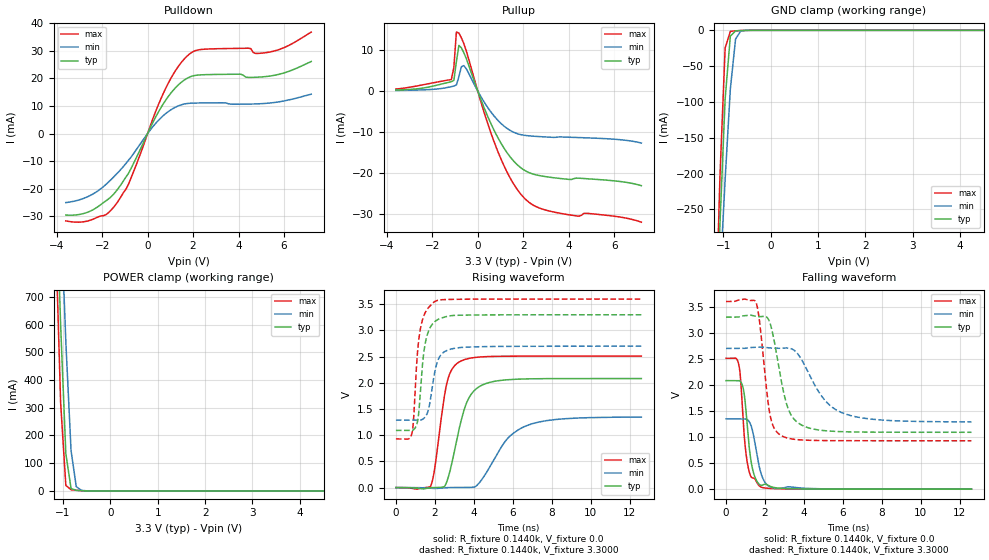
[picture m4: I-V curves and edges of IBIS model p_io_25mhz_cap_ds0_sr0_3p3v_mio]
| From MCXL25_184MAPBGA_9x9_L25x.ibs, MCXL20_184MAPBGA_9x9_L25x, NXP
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[Model] p_io_25mhz_cap_ds0_sr0_3p3v_mio
|   Model p_io_25mhz_cap_ds0_sr0_3p3v_mio
| This model was characterised for following simulation conditions:
| External (pad) voltage:
|   - Typ: 3.3V,   - Min: 2.7V,   - Max: 3.6V
| Library cells for typ/min/max conditions are connected as defined below:
|  pad - External Pad
|  ipp_do_lv - Core Input
|  ipp_obe_lv - Output Buffer Enable
|  IOGC - NC
|  REFH3V3 - REFH3V3
|  REFL3V3 - REFL3V3
|  ZI - NC
|  abut_ncal_vddio[1] - vddio
|  abut_ncal_vddio[2] - vddio
|  abut_ncal_vddio[3] - vssio
|  abut_ncal_vddio[4] - vddio
|  abut_ncal_vddio[5] - vddio
|  abut_ncal_vddio[6] - vssio
|  abut_pcal_vddio[1] - vssio
|  abut_pcal_vddio[2] - vssio
|  abut_pcal_vddio[3] - vddio
|  abut_pcal_vddio[4] - vssio
|  abut_pcal_vddio[5] - vssio
|  abut_pcal_vddio[6] - vddio
|  ipp_do_1p8v - ipp_do_1p8v
|  ipp_dse_lv - 0
|  ipp_eftd_lv - NC
|  ipp_ina_mux_vddio - NC
|  ipp_ina_mux_vddio[0] - NC
|  ipp_ina_mux_vddio[1] - NC
|  ipp_ina_r0_vddio - NC
|  ipp_ina_r0a_vddio - NC
|  ipp_ina_r0b_vddio - NC
|  ipp_ina_r0c_vddio - NC
|  ipp_ina_r0d_vddio - NC
|  ipp_ina_r0e_vddio - NC
|  ipp_ina_r0f_vddio - NC
|  ipp_ina_r300_vddio - NC
|  ipp_ina_r300a_vddio - NC
|  ipp_ina_r300b_vddio - NC
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Model_type I/O
Polarity   Non-Inverting
Enable   Active-High
Vinl =   0.9900V
Vinh =   2.3100V
Vmeas =  1.6500V
Cref =   30.0000pF
Rref =   1.0000M
Vref =   3.3000V
C_comp   1.2811pF   1.2304pF   1.3502pF
|C_comp_pullup   0.5379pF   0.5691pF   0.5166pF
|C_comp_pulldown   0.6571pF   0.6938pF   0.6279pF
[Model Spec]
| variable   typ   min   max
Vinh   2.3100V   1.8900V   2.5200V
Vinl   0.9900V   0.8100V   1.0800V
[Temperature Range]   25.0000   0.1250k   -40.0000
[Voltage Range]   3.3000V   2.7000V   3.6000V
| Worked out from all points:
|   slope of the pulldown table from 0 to 0.495 V, typ, clamps not added: 61.2 ohm
|   slope of the pullup table from 0 to 0.495 V, typ, clamps not added: 71.7 ohm
|   GND clamp passes 1 mA (typ) near -0.74 V on its own axis
|   POWER clamp passes 1 mA (typ) near -0.62 V on its own axis
|   rising waveform, R_fixture 0.1440k, V_fixture 0.0: 20-80 % time 844ps typ, 1.56ns min, 580ps max; typ from 0 V to 2.08 V
|   rising waveform, R_fixture 0.1440k, V_fixture 3.3000: 20-80 % time 369ps typ, 423ps min, 341ps max; typ from 1.09 V to 3.3 V
|   falling waveform, R_fixture 0.1440k, V_fixture 0.0: 20-80 % time 360ps typ, 440ps min, 328ps max; typ from 2.08 V to 0 V
|   falling waveform, R_fixture 0.1440k, V_fixture 3.3000: 20-80 % time 734ps typ, 1.47ns min, 472ps max; typ from 3.3 V to 1.09 V
[Pulldown]
|Voltage   I(typ)   I(min)   I(max)
-3.6V     -29.55mA   -25.02mA   -31.65mA
-2.5V     -28.03mA   -22.34mA   -31.35mA
-1.84V    -24.43mA   -18.49mA   -29.45mA
-1.4V     -21.05mA   -14.95mA   -25.71mA
-850mV    -14.55mA   -9.778mA   -18.52mA
800mV     12.15mA    7.264mA    16.46mA
1.35V     17.62mA    10.02mA    24.32mA
1.9V      20.65mA    11mA       29.17mA
4.43V     20.35mA    10.67mA    30.94mA
4.76V     20.41mA    10.74mA    29.03mA
5.31V     20.76mA    11.02mA    29.46mA
7.2V      26.12mA    14.27mA    36.78mA
[Pullup]
|Voltage   I(typ)   I(min)   I(max)
-3.6V     250.7uA    138.3uA    483.6uA
-1.16V    2.271mA    1.069mA    2.801mA
-1.05V    2.603mA    1.213mA    5.776mA
-940mV    7.093mA    1.465mA    14.38mA
-830mV    11.13mA    3.481mA    14.15mA
-720mV    10.55mA    5.904mA    12.99mA
-610mV    9.336mA    6.198mA    11.54mA
820mV     -10.68mA   -6.749mA   -13.84mA
1.48V     -16.43mA   -9.783mA   -21.75mA
2.03V     -19.25mA   -10.79mA   -26.01mA
3.35V     -21.16mA   -11.31mA   -29.53mA
7.2V      -23.09mA   -12.68mA   -32mA
[GND_clamp]
|Voltage   I(typ)   I(min)   I(max)
-3.6V     -5.309A    -4.128A    -6.876A
-1.18V    -466mA     -495.4mA   -458.9mA
-1.07V    -271.1mA   -348.5mA   -204.6mA
-960mV    -95.65mA   -207.9mA   -24.72mA
-850mV    -8.088mA   -81.85mA   -1.461mA
-740mV    -716.3uA   -12.13mA   -715.9uA
-630mV    -272.3uA   -921.7uA   -303uA
-300mV    -444.9nA   -2.656uA   -94.82nA
7.2V      0A         0A         0A
[POWER_clamp]
|Voltage   I(typ)   I(min)   I(max)
-3.6V     14.48A     12.95A     16.35A
-1.16V    1.177A     1.535A     951.2mA
-1.05V    598.4mA    1.032A     318mA
-940mV    134.2mA    537.3mA    20.05mA
-830mV    8.719mA    145.4mA    4.267mA
-720mV    2.135mA    15.38mA    2.236mA
-610mV    852.8uA    1.854mA    844.7uA
7.2V      0A         0A         0A
[Ramp]
| variable   typ   min   max
dV/dt_r  1.2492/0.8440n   0.8078/1.5631n   1.5061/0.5795n
dV/dt_f  1.3253/0.7337n   0.8457/1.4683n   1.6029/0.4716n
R_load = 0.1440k
[Rising Waveform]
R_fixture= 0.1440k
V_fixture= 0.0
V_fixture_min= 0.0
V_fixture_max= 0.0
|time   V(typ)   V(min)   V(max)
0s        4.636nV    156.4nV    15.8nV
1.788ns   -2.476mV   -13.22mV   30.75mV
1.985ns   614.7uV    -16.54mV   350mV
2.609ns   109.3mV    -732.9uV   1.985V
3.327ns   1.247V     1.006mV    2.415V
3.705ns   1.682V     1.312mV    2.463V
4.228ns   1.916V     68.95mV    2.491V
5.663ns   2.058V     907.7mV    2.509V
6.714ns   2.075V     1.183V     2.51V
12.6ns    2.082V     1.346V     2.51V
[Rising Waveform]
R_fixture= 0.1440k
V_fixture= 3.3000
V_fixture_min= 2.7000
V_fixture_max= 3.6000
|time   V(typ)   V(min)   V(max)
0s        1.091V     1.288V     928.5mV
809.1ps   1.091V     1.288V     1.016V
903.5ps   1.104V     1.288V     1.288V
1.053ns   1.188V     1.289V     2.297V
1.227ns   1.674V     1.289V     2.969V
1.503ns   2.75V      1.351V     3.342V
2.031ns   3.18V      2.273V     3.561V
2.397ns   3.245V     2.568V     3.588V
3.256ns   3.291V     2.673V     3.596V
12.6ns    3.3V       2.7V       3.6V
[Falling Waveform]
R_fixture= 0.1440k
V_fixture= 0.0
V_fixture_min= 0.0
V_fixture_max= 0.0
|time   V(typ)   V(min)   V(max)
0s        2.082V     1.348V     2.51V
621.3ps   2.083V     1.348V     2.437V
729.7ps   2.07V      1.348V     2.187V
840.7ps   1.99V      1.348V     1.54V
988.5ps   1.646V     1.349V     800.9mV
1.167ns   877.3mV    1.306V     364.3mV
1.415ns   307.4mV    1.023V     213.5mV
1.767ns   77.16mV    339.7mV    45.45mV
2.632ns   22.86mV    12.17mV    7.951mV
12.6ns    198.8nV    13.88uV    45.48nV
[Falling Waveform]
R_fixture= 0.1440k
V_fixture= 3.3000
V_fixture_min= 2.7000
V_fixture_max= 3.6000
|time   V(typ)   V(min)   V(max)
0s        3.3V       2.7V       3.6V
1.54ns    3.316V     2.722V     3.58V
1.721ns   3.308V     2.726V     3.214V
2.263ns   3.179V     2.707V     1.413V
2.866ns   2.02V      2.706V     1.021V
3.216ns   1.517V     2.705V     974.9mV
3.663ns   1.282V     2.603V     950mV
4.939ns   1.127V     1.77V      932.3mV
5.972ns   1.103V     1.463V     929.7mV
12.6ns    1.091V     1.29V      928.5mV
